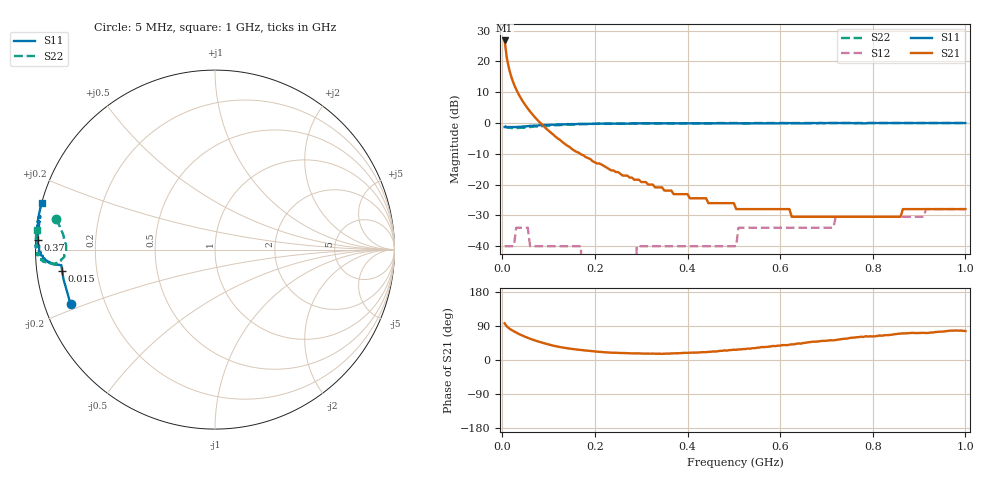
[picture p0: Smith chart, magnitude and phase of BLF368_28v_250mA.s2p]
! Filename:  BLF368_28v_250mA.s2p
! Philips part #: BLF368  !date: 21-05-2003
!28V @250 mA
!D:\Vee measurements\measurement data\VDMOST\BLF368\28v_250mA_#1
# HZ S MA R 50
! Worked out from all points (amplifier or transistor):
!   200 points, 5 MHz to 1 GHz, reference 50 ohm
!   highest |S21| = 26.8 dB at 5 MHz (marker M1)
!   |S21| within 3 dB of that: start of sweep to 7.548 MHz
!   S11 on the Smith chart (normalised r, x): 5 MHz: 0.08, -0.18; 15 MHz: 0.08, -0.07; 370 MHz: 0.01, +0.03; 1 GHz: -0.00, +0.13
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5000000  0.86 -159.2  21.94 96.8  0.01 -0.8  0.9 169.1
1e7  0.86 -168.9  11.14 88.5  0.01 21.1  0.85 174.3
1.5e7  0.86 -172.1  7.38 83.2  0.01 22.3  0.84 176.6
2e7  0.86 -173.4  5.45 79.2  0.01 18.7  0.83 178.2
2.5e7  0.86 -173.9  4.3 75.8  0.01 13.8  0.83 179.5
3e7  0.86 -174.2  3.53 72.3  0.02 8.7  0.83 -179.8
4e7  0.87 -174.4  2.54 66.3  0.02 0.3  0.84 -178.0
5.5e7  0.89 -174.6  1.72 58.5  0.02 -9.8  0.86 -176.2
6e7  0.9 -174.7  1.54 56.1  0.01 -12.5  0.86 -175.9
9.5e7  0.93 -175.7  0.81 42.6  0.01 -25.4  0.9 -175.0
1.7e8  0.97 -178.2  0.31 26.5  0.01 -23.1  0.96 -176.0
1.75e8  0.97 -178.4  0.3 25.8  0 -21.2  0.96 -176.1
2.85e8  0.98 178.7  0.12 17.5  0 66.3  0.99 -178.3
2.9e8  0.98 178.6  0.12 17.3  0.01 68.0  0.99 -178.4
3.4e8  0.99 177.5  0.09 16.6  0.01 76.5  0.99 -179.1
3.7e8  0.99 177.0  0.07 17.6  0.01 80.6  0.99 -179.5
5.05e8  0.99 174.3  0.04 26.8  0.01 88.4  1 178.8
5.1e8  0.99 174.2  0.04 27.8  0.02 88.5  1 178.8
6.7e8  1 171.3  0.03 48.4  0.02 90.7  1 177.1
7.2e8  1 170.5  0.03 52.8  0.03 91.1  1 176.7
8.35e8  1 168.3  0.03 65.8  0.03 93.2  1 175.6
1e9  1 165.1  0.04 76.4  0.04 92.3  1 173.8
